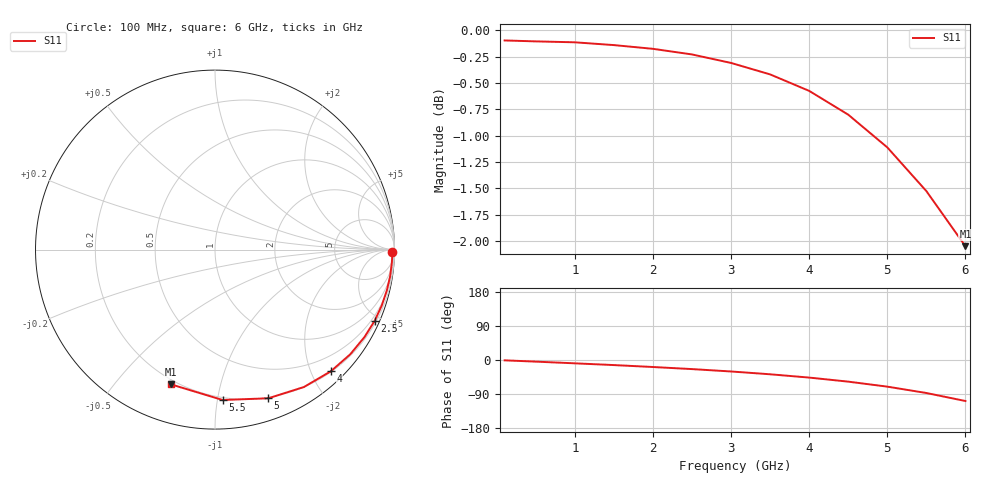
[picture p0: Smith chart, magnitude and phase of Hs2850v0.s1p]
!HSMS-2850 zero bias Schottky diode
!S-parameters at zero bias.  Last updated 6/7/94
# ghz s ma r 50
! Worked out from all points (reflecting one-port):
!   13 points, 100 MHz to 6 GHz, reference 50 ohm
!   lowest |S11| = -2.0 dB at 6 GHz (marker M1), VSWR 8.52, Z = 8.88 - j35.4 ohm
!   phase of S11 starts at -1 deg and turns -107 deg over the sweep
!   S11 on the Smith chart (normalised r, x): 100 MHz: open; 2.5 GHz: 0.30, -4.69; 4 GHz: 0.21, -2.32; 5 GHz: 0.19, -1.40; 5.5 GHz: 0.18, -1.04; 6 GHz: 0.18, -0.71
0.1  0.989 -0.9
0.5  0.988 -4.3
1  0.987 -8.8
1.5  0.984 -13.4
2  0.98 -18.5
2.5  0.974 -24.0
3  0.965 -30.3
3.5  0.953 -37.7
4  0.936 -46.4
4.5  0.912 -57.1
5  0.88 -70.3
5.5  0.839 -87.1
6  0.79 -108.2
